| TEXAS INSTRUMENTS INCORPORATED
| Standard Linear and Logic Group
| IBIS Model of TS5A23166
| 0.9-OHM DUAL SPST ANALOG SWITCH
| 5-V/3.3-V 2-CHANNEL ANALOG SWITCH
| This file contains package information for the following:
|  VSSOP 8-pin (DCU) package as [Component] TS5A23166_DCU
|  DSBGA 8-pin (YZP) package as [Component] TS5A23166_YZP
|  NanoFree WCSP 8-pin (YZT) package as [Component] TS5A23166_YZT
| This device can be powered at the following Vccs:
|  5 volt Vcc
|  3.3 volt Vcc
|  2.5 volt Vcc
|  1.8 volt Vcc
| This file provides unique models under the [Model Selector] for each Vcc.
| For operation at a specific Vcc, select the appropriate model after each
| [Model Selector] keyword.
[IBIS Ver]   3.2
[Comment char]  |_char
[File Name]   ts5a23166.ibs
[File Rev]   1.1 | x_die
[Date]   April 8, 2005
[Source]   Data created from TI-SPICE simulations at TI-SLL.
[Notes]   The following is an IBIS list for the TS5A23166.
   Please contact sllibis@ti.com with questions and
   comments concerning SLL IBIS models.
   - FILE REV HISTORY
   - 1.1 Release IBIS file on 08/24/07
   - Power clamp data deleted in the IN models as there
   is no power-clamp diode.
   - Non-monotonic data due to FET characteristics.
   - NCH & PCH MOSFETS, so [Series Mosfet] model can have rising
   or falling currents
[Disclaimer] Property of Texas Instruments Incorporated.  Unauthorized
   reproduction and/or distribution is strictly prohibited.
   This product is protected under copyright law.
   Created  2005, (C) Copyright  2005, Texas Instruments
   Incorporated, All Rights Reserved
   UNLESS THERE IS A SIGNED, WRITTEN AGREEMENT TO THE
   CONTRARY, TEXAS INSTRUMENTS (TI) IS PROVIDING THE IBIS
   MODELS  AND WITHOUT ANY WARRANTY, EXPRESSED OR
   IMPLIED.  TI assumes no liability for:
   1) the accuracy of the IBIS models provided to your
   company;
   2) the proper functioning of these IBIS Models in your
   design or for any resulting applications; or
   3) infringement of patents, copyrights or intellectual
   property rights resulting from your use of these IBIS
   models.
   TI provides IBIS Models as a service to our customers.
   You and your company shall not distribute, sell or give
   these models to anyone else without prior written
   permission from TI.
   TI reserves the right to make changes to our products or
   to discontinue any semiconductor product or service
   without notice, and advises our customers to obtain the
   latest version of relevant information to verify, before
   placing orders, that the information being relied on is
   current.
   Please be aware that your receipt and use of the IBIS
   information provided shall serve as acceptance of these
   terms and conditions.  If you do not accept these terms,
   you should return or destroy the IBIS models and any
   other accompanying information immediately.
| Component TS5A23166_DCU 8-pin TSSOP
[Component]   TS5A23166_DCU
[Manufacturer]   Texas Instruments, Inc.
[Package]
|   typ   min   max
R_pkg   1.400e-02   1.300e-02   1.500e-02
L_pkg   1.289e-09   1.025e-09   2.014e-09
C_pkg   1.360e-13   6.600e-14   2.940e-13
[Pin]   signal_name   model_name   R_pin   L_pin   C_pin
1   NO1   TS5A23166_COM   1.400e-02   1.387e-09   1.760e-13
2   COM1   TS5A23166_NO   1.300e-02   1.026e-09   6.600e-14
3   IN2   TS5A23166_IN   1.300e-02   1.032e-09   6.700e-14
4   GND   GND   1.500e-02   2.014e-09   2.940e-13
5   NO2   TS5A23166_COM   1.400e-02   1.412e-09   1.780e-13
6   COM2   TS5A23166_NO   1.300e-02   1.030e-09   6.600e-14
7   IN1   TS5A23166_IN   1.300e-02   1.025e-09   6.600e-14
8   VCC   POWER   1.400e-02   1.386e-09   1.760e-13
| Component TS5A23166_YZP 8-pin NanoFree WCSP
[Component]   TS5A23166_YZP
[Manufacturer]   Texas Instruments, Inc.
[Package]
|   typ   min   max
R_pkg   0.001   0.001   0.001
L_pkg   0.021nH   0.021nH   0.021nH
C_pkg   0.043pF   0.042pF   0.044pF
[Pin]   signal_name   model_name   R_pin   L_pin   C_pin
1   NO1   TS5A23166_COM   0.046   2.861nH   0.321pF
2   COM1   TS5A23166_NO   0.037   2.437nH   0.286pF
3   IN2   TS5A23166_IN   0.034   2.419nH   0.286pF
4   GND   GND   0.043   2.784nH   0.321pF
5   NO2   TS5A23166_COM   0.043   2.784nH   0.321pF
6   COM2   TS5A23166_NO   0.035   2.420nH   0.286pF
7   IN1   TS5A23166_IN   0.037   2.437nH   0.286pF
8   VCC   POWER   0.046   2.860nH   0.321pF
| Component TS5A23166_YZT 8-pin NanoFree WCSP
[Component]   TS5A23166_YZT
[Manufacturer]   Texas Instruments, Inc.
[Package]
|   typ   min   max
R_pkg   0.001   0.001   0.001
L_pkg   0.021nH   0.021nH   0.021nH
C_pkg   0.043pF   0.042pF   0.044pF
[Pin]   signal_name   model_name   R_pin   L_pin   C_pin
1   NO1   TS5A23166_COM   0.046   2.861nH   0.321pF
2   COM1   TS5A23166_NO   0.037   2.437nH   0.286pF
3   IN2   TS5A23166_IN   0.034   2.419nH   0.286pF
4   GND   GND   0.043   2.784nH   0.321pF
5   NO2   TS5A23166_COM   0.043   2.784nH   0.321pF
6   COM2   TS5A23166_NO   0.035   2.420nH   0.286pF
7   IN1   TS5A23166_IN   0.037   2.437nH   0.286pF
8   VCC   POWER   0.046   2.860nH   0.321pF
[Series Switch Groups]
| Function Group States
On  1 /   | COM1->NO1 IN1 HIGH
On  2 /   | COM2->NO2 IN2 HIGH
On  3 /   | NO1->COM1 IN1 HIGH
On  4 /   | NO2->COM2 IN2 HIGH
Off 1 3 /   | IN1 LOW
Off 2 4  /   | IN2 LOW
[Series Pin Mapping]   pin_2   model_name   function_table_group
1   2   TS5A23166_COM_50_S   1
| 1   2   TS5A23166_COM_33_S   1
| 1   2   TS5A23166_COM_25_S   1
| 1   2   TS5A23166_COM_18_S   1
5   6   TS5A23166_COM_50_S   2
| 5   6   TS5A23166_COM_33_S   2
| 5   6   TS5A23166_COM_25_S   2
| 5   6   TS5A23166_COM_18_S   2
2   1   TS5A23166_NO_50_S   3
| 2   1   TS5A23166_NO_33_S   3
| 2   1   TS5A23166_NO_25_S   3
| 2   1   TS5A23166_NO_18_S   3
6   5   TS5A23166_NO_50_S   4
| 6   5   TS5A23166_NO_33_S   4
| 6   5   TS5A23166_NO_25_S   4
| 6   5   TS5A23166_NO_18_S   4
| Model TS5A23166_IN
[Model Selector]   TS5A23166_IN
TS5A23166_IN_50   5 volt Vcc
TS5A23166_IN_33   3.3 volt Vcc
TS5A23166_IN_25   2.5 volt Vcc
TS5A23166_IN_18   1.8 volt Vcc
| Model TS5A23166_COM
[Model Selector]   TS5A23166_COM
TS5A23166_COM_50   5 volt Vcc
TS5A23166_COM_33   3.3 volt Vcc
TS5A23166_COM_25   2.5 volt Vcc
TS5A23166_COM_18   1.8 volt Vcc
| Model TS5A23166_COM_S
[Model Selector]   TS5A23166_COM_S
TS5A23166_COM_50_S   5 volt Vcc
TS5A23166_COM_33_S   3.3 volt Vcc
TS5A23166_COM_25_S   2.5 volt Vcc
TS5A23166_COM_18_S   1.8 volt Vcc
| Model TS5A23166_NO
[Model Selector]   TS5A23166_NO
TS5A23166_NO_50   5 volt Vcc
TS5A23166_NO_33   3.3 volt Vcc
TS5A23166_NO_25   2.5 volt Vcc
TS5A23166_NO_18   1.8 volt Vcc
| Model TS5A23166_NO_S
[Model Selector]   TS5A23166_NO_S
TS5A23166_NO_50_S   5 volt Vcc
TS5A23166_NO_33_S   3.3 volt Vcc
TS5A23166_NO_25_S   2.5 volt Vcc
TS5A23166_NO_18_S   1.8 volt Vcc
[Model]   TS5A23166_COM_50_S
Model_type  Series_switch
| variable   typ   min   max
C_comp   0   0   0
[Temperature Range]   40   100   -40
| Ambient temperature   25   85   -40
[Voltage range]   5   4.5   5.5
[On]
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[Off]
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[Model]   TS5A23166_COM_33_S
Model_type  Series_switch
| variable   typ   min   max
C_comp   0   0   0
[Temperature Range]   40   100   -40
| Ambient temperature   25   85   -40
[Voltage range]   3.3   3   3.6
[On]
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[Off]
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[Model]   TS5A23166_COM_25_S
Model_type  Series_switch
| variable   typ   min   max
C_comp   0   0   0
[Temperature Range]   40   100   -40
| Ambient temperature   25   85   -40
[Voltage range]   2.5   2.3   2.7
[On]
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[Off]
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[Model]   TS5A23166_COM_18_S
Model_type  Series_switch
| variable   typ   min   max
C_comp   0   0   0
[Temperature Range]   40   100   -40
| Ambient temperature   25   85   -40
[Voltage range]   1.8   1.65   1.95
[On]
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[Off]
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[Model]   TS5A23166_NO_50_S
Model_type  Series_switch
| variable   typ   min   max
C_comp   0   0   0
[Temperature Range]   40   100   -40
| Ambient temperature   25   85   -40
[Voltage range]   5   4.5   5.5
[On]
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[Off]
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[Model]   TS5A23166_NO_33_S
Model_type  Series_switch
| variable   typ   min   max
C_comp   0   0   0
[Temperature Range]   40   100   -40
| Ambient temperature   25   85   -40
[Voltage range]   3.3   3   3.6
[On]
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[Off]
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[Model]   TS5A23166_NO_25_S
Model_type  Series_switch
| variable   typ   min   max
C_comp   0   0   0
[Temperature Range]   40   100   -40
| Ambient temperature   25   85   -40
[Voltage range]   2.5   2.3   2.7
[On]
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[Off]
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[Model]   TS5A23166_NO_18_S
Model_type  Series_switch
| variable   typ   min   max
C_comp   0   0   0
[Temperature Range]   40   100   -40
| Ambient temperature   25   85   -40
[Voltage range]   1.8   1.65   1.95
[On]
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[Off]
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| Models and submodels in the file (20): TS5A23166_IN_50 (Input), TS5A23166_IN_33 (Input), TS5A23166_IN_25 (Input), TS5A23166_IN_18 (Input), TS5A23166_COM_50_S (Series_switch), TS5A23166_COM_50 (Terminator), TS5A23166_COM_33_S (Series_switch), TS5A23166_COM_33 (Terminator), TS5A23166_COM_25_S (Series_switch), TS5A23166_COM_25 (Terminator), TS5A23166_COM_18_S (Series_switch), TS5A23166_COM_18 (Terminator), TS5A23166_NO_50_S (Series_switch), TS5A23166_NO_50 (Terminator), TS5A23166_NO_33_S (Series_switch), TS5A23166_NO_33 (Terminator), TS5A23166_NO_25_S (Series_switch), TS5A23166_NO_25 (Terminator), TS5A23166_NO_18_S (Series_switch), TS5A23166_NO_18 (Terminator)
